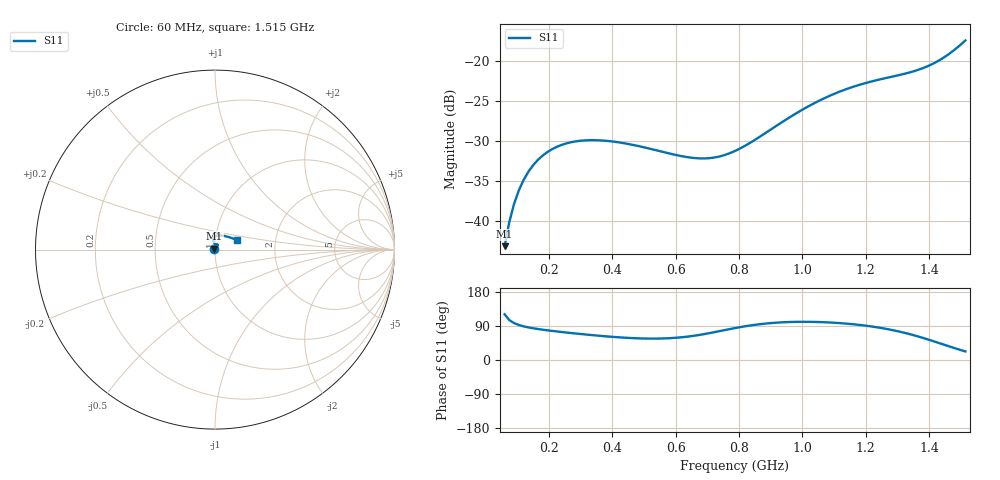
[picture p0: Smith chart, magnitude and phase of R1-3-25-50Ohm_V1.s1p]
!version-1
!date-08.2020
!Series
#	GHZ S RI R 50.0
!	FREQ.GHZ	S11RE	S11IM
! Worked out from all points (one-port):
!   98 points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, 60 MHz to 1.515 GHz, reference 50 ohm
!   lowest |S11| = -43.2 dB at 60 MHz (marker M1), VSWR 1.01, Z = 49.6 + j0.591 ohm
!   |S11| at or under -10 dB: start of sweep to end of sweep
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0.06  -0.00352 0.00595
0.075  -0.00259 0.00948
0.09  -0.00162 0.0126
0.105  -0.000628 0.0155
0.12  0.000379 0.018
0.135  0.0014 0.0202
0.15  0.00242 0.0221
0.18  0.00444 0.0252
0.21  0.00641 0.0273
0.255  0.00916 0.0291
0.33  0.0129 0.0292
0.375  0.0145 0.0282
0.435  0.0157 0.0263
0.615  0.0129 0.022
0.66  0.0107 0.0222
0.705  0.00817 0.0232
0.75  0.0053 0.0251
0.795  0.00223 0.0277
0.84  -0.000869 0.0312
0.975  -0.00849 0.0456
1.065  -0.00988 0.0571
1.155  -0.00572 0.0682
1.245  0.00661 0.0765
1.335  0.0301 0.079
1.38  0.0471 0.077
1.425  0.0682 0.0722
1.47  0.0938 0.0639
1.515  0.1245 0.0518
